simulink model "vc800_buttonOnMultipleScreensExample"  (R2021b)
settings: Solver=FixedStepDiscrete  StartTime=0.0  StopTime=10.0  FixedStep=0.01  RelTol=1e-3  EnableMultiTasking=on
PreLoadFcn:
  | try, model_open; catch, disp('Error occurred while executing model pre-load callback: model_open.m'); disp('Please assure that the MATLAB working directory is set to the model directory before opening.'); end
InitFcn:
  | try, model_open; catch, end
model workspace (MAT data in the model file):
  IOScreen_Label_XCoord = 1
  IOScreen_Row1_YCoord = 1
  IOScreen_Row2_YCoord = 12
  IOScreen_Value_XCoord = 110
  MainScreen_Row1_YCoord = 7
  MainScreen_Row2_YCoord = 23
  MainScreen_Symbols_XCoord = 1
  MainScreen_Units_XCoord = 69
  MainScreen_Value_XCoord = 64
undefined symbols (not defined in the file or in its folder): case, curr_screen, default, DISP, filtering, gesture, hex2dec, Mode, No, raptor_get_buildNum, raptor_get_safe_string, raptor_hwexp, raptor_xcp_function, Screens, VC800, Voltage
libraries: Raptor_display_lib x190, Raptor_lib x97, simulink_extras x11, Raptor_Datalogging_lib x10, simulink x2
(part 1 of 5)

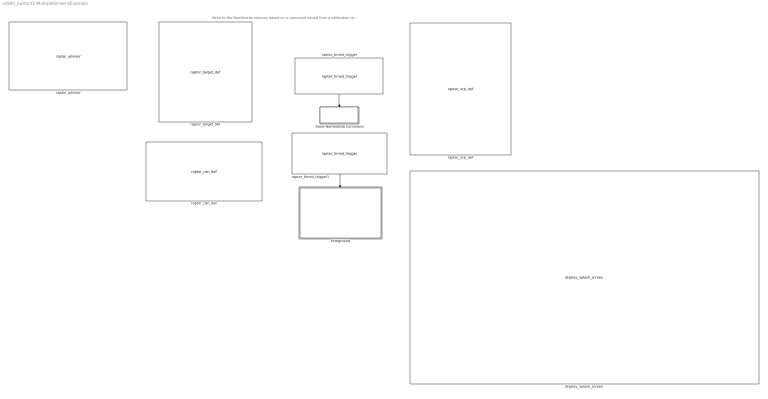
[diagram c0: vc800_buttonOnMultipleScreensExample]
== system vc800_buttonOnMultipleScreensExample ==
  note: Write to the NonVolatile memory based on a command issued from a calibration tool. This display does not have an option for a controlled shutdown but too many writes will burn out the internal NonVolatile memory.
  Foreground : Subsystem
  Store NonVolatile Command : Subsystem  TreatAsAtomicUnit=on
  display_splash_screen : Raptor_display_lib/Screen Functions/display_splash_screen  ImageFile=background_newsplash.bmp
  raptor_advisor : Raptor_lib/Configuration/raptor_advisor  pop_setEnable=Enable All  ckb_Raptor=on  ckb_AppMonitor=on  tbl_AppMonitor={ 'on', 'App Monitor'; 'on', 'App Monitor Measurement'; 'on', 'App Monitor Stop'; 'on', 'Reboot'; 'on', 'Task Monitor'; 'on', 'Task Monitor Measurement' }  ckb_CAN=on  tbl_CAN="{ 'on', 'CAN Baud Rate'; 'on', 'CAN Bus Off Recovery'; 'on', 'CAN Definition'; 'on', 'CAN Hardware Mailbox Config'; 'on', 'CAN Mailbox Properties'; 'on', 'CAN Partial Networking'; 'on', 'CAN Queue Info'; 'on', 'CAN Rx Message'; 'on', 'CAN Rx Raw'; 'on', 'CAN State'; 'on', 'CAN Trigger'; 'on', 'CAN Tx Message'; 'on', 'CAN Tx Raw'; 'on', 'CAN/FD Definition'; 'on', 'CAN/FD Rx Message'; 'on', 'CAN/FD 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"  ckb_Checksum=on  tbl_Checksum={ 'on', 'Calculate Checksum'; 'on', 'Read Checksum' }  ckb_Config=on  tbl_Config={ 'on', 'Configuration Read'; 'on', 'System Variable Access Level'; 'on', 'ECU Definition'; 'on', 'Set Target Address'; 'on', 'XCP Custom Security Seed/Key'; 'on', 'XCP Custom Security Trigger'; 'on', 'XCP Protocol Definition'; 'on', 'XCP Query'; 'on', 'XCP Set Address' }  ckb_DataStore=on  tbl_DataStore={ 'on', 'Adjustment'; 'on', 'Data Store'; 'on', 'Data Read'; 'on', 'Data Write'; 'on', 'Load NonVolatile Defaults'; 'on', 'Fixed NV Manager'; 'on', 'Measurement'; 'on', 'Memory Read'; 'on', 'NonVolatile Settings'; 'on', 'Override'; 'on', 'Fixed NonVolatile Status'; 'on', 'NonVolatile Status'; 'on', 'Store NonVolatile' }  ckb_Engine=on  tbl_Engine={ 'on', 'Angle Time'; 'on', 'CamShaft Sensor Info'; 'on', 'Encoder Def'; 'on', 'Injector Output'; 'on', 'Knock Results'; 'on', 'Knock Input'; 'on', 'Spark Output'; 'on', 'Wideband O2 Input' }  ckb_Ethernet=on  tbl_Ethernet="{ 'on', 'Ethernet Adapter Get MAC Address'; 'on', 'Ethernet Definition'; 'on', 'Ethernet Interface Definition'; 'on', 'Ethernet Interface Get VLAN'; 'on', 'Ethernet Interface Set VLAN'; 'on', 'Ethernet Socket - TCP Server'; 'on', 'Ethernet Socket - UDP Server'; 'on', 'Ethernet Socket State'; 'on', 'Ethernet TCP Accept'; 'on', 'Ethernet TCP Close'; 'on', 'Ethernet TCP Connect'; 'on', 'Ethernet TCP 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"  ckb_OBD_Faults=on  tbl_OBD_Faults={ 'on', 'OBD Counter'; 'on', 'Increment OBD Counter'; 'on', 'Read OBD Counter'; 'on', 'Reset OBD Counter'; 'on', 'Drive Cycle Complete'; 'on', 'OBD Ratio'; 'on', 'Increment OBD Ratio'; 'on', 'Read OBD Ratio'; 'on', 'Reset OBD Ratio' }  ckb_Faults=on  tbl_Faults={ 'on', 'Fault Action'; 'on', 'Fault Action Iterator'; 'on', 'Fault Action Read'; 'on', 'Clear Fault'; 'on', 'Fault Data'; 'on', 'Fault Data Read'; 'on', 'Fault Data Write'; 'on', 'Fault'; 'on', 'Fault Handle'; 'on', 'Fault Iterator'; 'on', 'Fault Manager'; 'on', 'Fault Measurement'; 'on', 'Null Fault'; 'on', 'Fault Config'; 'on', 'Fault Reference'; 'on', 'Set Fault State'; 'on', 'Fault State Iter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  ckb_IO=on  tbl_IO={ 'on', 'Analog Input'; 'on', 'Analog Input Reference'; 'on', 'Analog Output'; 'on', 'Device Diagnostics'; 'on', 'Digital Input'; 'on', 'Digital Output'; 'on', 'Frequency Input'; 'on', 'H-Bridge Output'; 'on', 'IMU Calibrate'; 'on', 'IMU Reset'; 'on', 'IMU Status'; 'on', 'Inertial Measurement'; 'on', 'Input Capture Defn'; 'on', 'Input Capture Get'; 'on', 'Input Capture Trigger'; 'on', 'Input Statu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  ckb_LIN=on  tbl_LIN={ 'on', 'LIN Master Definition'; 'on', 'LIN Get Schedule'; 'on', 'LIN Rx Message'; 'on', 'LIN Set Schedule'; 'on', 'LIN Slave Definition'; 'on', 'LIN State'; 'on', 'LIN Trigger'; 'on', 'LIN Tx Message' }  ckb_SENT=on  tbl_SENT={ 'on', 'SENT Definition'; 'on', 'SENT Receive State' }  ckb_Serial=on  tbl_Serial={ 'on', 'Serial Definition'; 'on', 'Serial Rx'; 'on', 'Serial Trigger'; 'on', 'Serial Tx' }  ckb_Strings=on  tbl_Strings={ 'on', 'String'; 'on', 'Arr 2 Str'; 'on', 'String Length'; 'on', 'Printf'; 'on', 'String Reference'; 'on', 'scanf'; 'on', 'Str 2 Arr' }  ckb_Tables=on  tbl_Tables={ 'on', 'Table Adapt'; 'on', 'Axis'; 'on', 'Axis Reference'; 'on', 'Table Interpolate 1D'; 'on', 'Table Interpolate 1D Reference'; 'on', 'Table Interpolate 2D'; 'on', 'Table Interpolate 2D Reference' }  ckb_Time=on  tbl_Time={ 'on', 'Datetime Conversion In'; 'on', 'Datetime Conversion Out'; 'on', 'Real Time Clock Read'; 'on', 'Real Time Clock Set' }  ckb_Triggers=on  tbl_Triggers={ 'on', 'App Trigger'; 'on', 'dT'; 'on', 'Distributed Action Defn'; 'on', 'Distributed Action Execute'; 'on', 'Distributed Action Trigger'; 'on', 'Shutdown'; 'on', 'Sleep'; 'on', 'Startup'; 'on', 'Time'; 'on', 'Timed Trigger'; 'on', 'Timed Trigger Config'; 'on', 'Define Trigger'; 'on', 'Trigger Execute'; 'on', 'Output Trigger Reference'; 'on', 'Trigger Select' }  ckb_DataLog=on  tbl_DataLog={ 'on', 'Data Log Erase'; 'on', 'Data Log Read'; 'on', 'Data Log Write'; 'on', 'File Close'; 'on', 'File EOF'; 'on', 'File Exists'; 'on', 'File Get Free Space'; 'on', 'File Open'; 'on', 'File Position'; 'on', 'File Read'; 'on', 'File Remove'; 'on', 'File Rename'; 'on', 'File Seek'; 'on', 'File Size'; 'on', 'File Sync'; 'on', 'USB Eject'; 'on', 'USB Status'; 'on', 'File Write' }  ckb_Display=on  ckb_Drawing=on  tbl_Drawing={ 'on', 'Clear Rect'; 'on', 'Clear Screen'; 'on', 'Draw Arc'; 'on', 'Draw Button'; 'on', 'Draw Circle'; 'on', 'Draw Image'; 'on', 'Draw Line'; 'on', 'Draw Polygon'; 'on', 'Draw Rectangle'; 'on', 'Draw Text'; 'on', 'Element'; 'on', 'Fill Circle'; 'on', 'Fill Ellipse'; 'on', 'Fill Polygon'; 'on', 'Fill Rect'; 'on', 'Image Ref' }  ckb_Menu=on  tbl_Menu={ 'on', 'Menu Screen Definition'; 'on', 'Menu Sel Item'; 'on', 'Menu Text'; 'on', 'Menu Title' }  ckb_Prefab=on  tbl_Prefab={ 'on', 'Gauge: Create'; 'on', 'Gauge: Update' }  ckb_ScreenFuncs=on  tbl_ScreenFuncs={ 'on', 'Hide Buttonbar'; 'on', 'Button Bar Properties'; 'on', 'Setup Button'; 'on', 'Goto Screen'; 'on', 'Recalibrate Screen'; 'on', 'Screen Definition'; 'on', 'Screen Reference'; 'on', 'Screen Select'; 'on', 'Splash Screen' }  ckb_Touchscreen=on  tbl_Touchscreen={ 'on', 'Button Status'; 'on', 'Display Touchscreen'; 'on', 'Button Def'; 'on', 'Hot Area Actions'; 'on', 'Update Swipe Action' }  ckb_Modbus=on  tbl_Modbus={ 'on', 'Modbus Master'; 'on', 'Modbus Slave'; 'on', 'Modbus Slave Error'; 'on', 'Modbus Slave Response' }  ckb_Routing=on  tbl_Routing={ 'on', 'J1939 Message Router'; 'on', 'Message Hardware Filter'; 'on', 'Message Network'; 'on', 'Message Router' }  ckb_Safe=on  tbl_Safe={ 'on', 'Raptor Stack Check' }  ckb_J1939=on  ckb_DMA=on  tbl_DMA={ 'on', 'DM14/15/16 Definition: DM14 Rx'; 'on', 'DM14/15/16 Definition: DM15 Rx'; 'on', 'DM14/15/16 Definition: DM15 Tx'; 'on', 'DM14/15/16 Definition: DMA Manager'; 'on', 'DMA Address Space Definition'; 'on', 'DMA Address Space Return'; 'on', 'DMA Address Space Trigger'; 'on', 'DMA Key'; 'on', 'DMA Key Trigger' }  ckb_DM_Msgs=on  tbl_DM_Msgs={ 'on', 'DM4 Transmit'; 'on', 'DM5 Transmit'; 'on', 'DM8 Transmit'; 'on', 'DM19 Transmit'; 'on', 'DM20 Transmit'; 'on', 'DM21 Transmit'; 'on', 'DM22 Rx Trigger'; 'on', 'DM24 Transmit'; 'on', 'DM25 Transmit'; 'on', 'DM26 Transmit'; 'on', 'DM29 Transmit'; 'on', 'DM30 Transmit'; 'on', 'DM33 Transmit'; 'on', 'DM34 Transmit'; 'on', 'DTC Transmit' }  ckb_EFF=on  tbl_EFF={ 'on', 'Clear Expanded FF'; 'on', 'Write Expanded FF'; 'on', 'Expanded FF Status' }  ckb_PGN_Tx=on  tbl_PGN_Tx={ 'on', 'CBI Transmit'; 'on', 'CI Transmit'; 'on', 'EC1 Transmit'; 'on', 'ECUID Transmit'; 'on', 'GTFI Transmit'; 'on', 'LTFI Transmit'; 'on', 'RC Transmit'; 'on', 'SOFT Transmit'; 'on', 'TTI2 Transmit'; 'on', 'VI Transmit' }  ckb_SPN=on  tbl_SPN={ 'on', 'SPN Read'; 'on', 'SPN Write' }  ckb_J1939_TP=on  tbl_J1939_TP={ 'on', 'J1939 DTC Rx Handler'; 'on', 'Source Addr'; 'on', 'PGN Enable'; 'on', 'PGN Request Slot'; 'on', 'PGN Enable'; 'on', 'PGN Trigger'; 'on', 'Tx ACK/NACK'; 'on', 'J1939 Protocol'; 'on', 'J1939 Transport Protocol Receive'; 'on', 'PGN Rx Trigger' }  ckb_UDS=on  ckb_ISO14229=on  tbl_ISO14229={ 'on', 'ISO14229 Custom Service 0x31'; 'on', 'ISO14229 Service 0x10 - Session Control'; 'on', 'ISO14229 Service 0x11 - ECU Reset'; 'on', 'ISO14229 Service 0x14 - Clear Diagnostic Information'; 'on', 'ISO14229 Service 0x19 - Read DTC Information'; 'on', 'ISO14229 Service 0x19 - Extended Data Definition'; 'on', 'ISO14229 Service 0x19 - Snapshot Record Definition'; 'on', 'ISO14229 Service 0x19 - Sna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  ckb_ISO15031=on  tbl_ISO15031={ 'on', 'ISO15031 Custom Service'; 'on', 'ISO15031 Service 0x01'; 'on', 'ISO15031 Service 0x03 - Emission-related diagnostic trouble codes'; 'on', 'ISO15031 Service 0x04 - Clear Diagnostic Information'; 'on', 'ISO15031 Service 0x07 - Emission-related pending diagnostic trouble codes'; 'on', 'ISO15031 Service 0x09 - Calibration Identification'; 'on', 'ISO15031 Service 0x09 - Calibration Verificatio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  ckb_ISO15765=on  tbl_ISO15765={ 'on', 'ISO15765 Protocol Receive Queue Info'; 'on', 'ISO15765 Protocol Transmit Queue Info'; 'on', 'ISO15765 Protocol Transmit Raw' }  ckb_UDS_Basics=on  tbl_UDS_Basics={ 'on', 'UDS Client Functional Address Request'; 'on', 'UDS Protocol Client Request Raw'; 'on', 'UDS Protocol Receive Raw'; 'on', 'UDS Server Service Process Raw'; 'on', 'UDS Protocol Transmit Raw' }  ckb_UDS_Other=on  tbl_UDS_Other={ 'on', 'UDS Protocol'; 'on', 'UDS Set Buffer Storage' }
  raptor_can_def : Raptor_lib/CAN/raptor_can_def  canBus='CAN1'  resourceValues=CAN1|(None)  resource=CAN1  baudRateValues=125k|250k|500k|1000k  baudRate=250k  enable_baud_rate_config=0  sim_func_name='ConfigureCANBaudRate'  createButton=[]  txQueueSize=16  rxQueueSize=16  useCustomBR=0  customBR='CustomBaudRate'  updateButton=[]
  raptor_target_def : Raptor_lib/Configuration/raptor_target_def  targetValues=DISP-VC128-1901|DISP-VC320L-1402|DISP-VC320-1204|DISP-VC800-1402|DISP-VC500-1904|DISP-VC700-2003|DISP-VC300R-2004|GCM-5634M-070-1559|GCM-5634M-070-1562|ECM-1793-196-1503|GCM-1793-196-1503|GCM-5605B-048-1906|GCM-5605B-048-2104|RCM-5743R-080-2005|RCM-5743R-080-2106|RCM-5743R-080-2203|RCM-5743R-080-2304|UAS-5743R-047-2102|UAS-5743R-047-2107|EOL-58NN-176-2204|RCM-58NN-112-2103|RCM-58NN-112-2202|RCM-58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  target=DISP-VC800-1402  simpack=0  simulator=1  heap=2*1024  stack=2*1024  fgndStack=2*1024  bgndStack=2*1024  idleStack=1024  intStack=1536  sdStack=1024  appStack=1024  ecuaddr=253  uds_server_addr_ext=0  uds_server_addr=hex2dec('600')  uds_client_addr=hex2dec('650')  callocValues=Constant (FLASH)|NonVolatile (EEPROM)  calloc=NonVolatile (EEPROM)  compilerValues=Device:arm-2014.05_1.0.0 Simulator:None (disabled)|Device:arm-2014.05_1.0.0 Simulator:Visual Studio Community 2017  compiler=Device:arm-2014.05_1.0.0 Simulator:Visual Studio Community 2017  setFileName=1  exeName=[raptor_get_safe_string(bdroot) '_']  addBuildNum=1  minVerChars=3  extraOutput=0  buildLocationValues=Raptor Default|Model Directory|User Defined  buildLocation=Raptor Default  exeLocation=''  exeFileButton=0  a2lLocation=''  a2lFileButton=0  rpgLocation=''  rpgFileButton=0
  raptor_timed_trigger : Raptor_lib/Triggers/raptor_timed_trigger  triggerValues=Foreground|Foregroundx2|Foregroundx5|Foregroundx10|Foregroundx50|Background|Backgroundx2|Backgroundx5|Backgroundx10|Backgroundx20|Second|Minute  trigger=Background  inherited=0  alwaysEnabled=1  triggerPriority=0  triggerName=BGND_kLoVr
  raptor_timed_trigger1 : Raptor_lib/Triggers/raptor_timed_trigger  triggerValues=Foreground|Foregroundx5|Foregroundx10|Foregroundx50|Second|Minute  trigger=Foreground  inherited=0  alwaysEnabled=1  triggerPriority=0  triggerName=7Je7r
  raptor_xcp_def : Raptor_lib/Configuration/raptor_xcp_def  XCPname='XCP1'  canBus='CAN1'  bcID=hex2dec('100')  bcID_TypeValues=Standard|Extended  bcID_Type=Standard  rxID=hex2dec('200')  rxID_TypeValues=Standard|Extended  rxID_Type=Standard  txID=hex2dec('300')  txID_TypeValues=Standard|Extended  txID_Type=Standard  daqRates=[10 100]  numODTs=20  genCANAPE=0  genVISION=0  securityValues=Standard|None|Custom User Defined|MH_SB_4  security=Standard  dllName=raptor_XCPSecurity.dll  accessValues=4|3|2|1  access=1  bcStorageValues=[]  bcStorage=Calibration  txStorageValues=[]  txStorage=Calibration  rxStorageValues=[]  rxStorage=Calibration
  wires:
  raptor_timed_trigger1/1 -> Foreground/Trigger
  raptor_timed_trigger/1 -> Store NonVolatile Command/Trigger

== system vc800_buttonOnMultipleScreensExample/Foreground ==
  Trigger : TriggerPort  TriggerType=function-call  VariantControl=Variant  PortDimensions=1
  Display : Subsystem
  Plant : Subsystem
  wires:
  Display/1(Actuators) -> Plant/1(Actuators)
  Plant/1(Sensors) -> Display/1(Sensors)

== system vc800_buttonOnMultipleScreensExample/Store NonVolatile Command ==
  note: Setting the StoreNonvolatileCommand value to to 1 in the calibration tool will cause this subsystem to execute, calling the 'Store Nonvolatile' function. The StoreNonvolatileCommand value will be set to 0 inside the subsytem so that the Store event happens once.
  function : TriggerPort  TriggerType=function-call  VariantControl=Variant
  Store NV : Subsystem  TreatAsAtomicUnit=on
  raptor_data_def : Raptor_lib/Data Storage/raptor_data_def  dataName='StoreNonVolatileCommand'  initValue=false  dataType=boolean  storage=Volatile (RAM)  calVisible=on  calType=Adjustment  calDispType=Enumeration  calEnum={'Not Writing', 'Start Write'}  calGain=1.0  calOffset=0  calMin=-inf  calMax=inf  calFormat='-1'  calUnit=''  calHelp=''  calAccess=1  calFunction=raptor_xcp_function(gcb)  calDispHeaders=off  calColHeaders={'Col1' 'Col2' 'Col3'}  calRowHeaders={'Row1' 'Row2' 'Row3'}
  raptor_data_read : Raptor_lib/Data Storage/raptor_data_read  dataName='StoreNonVolatileCommand'  dataShape=Scalar  idxSource=Input  idxRow=1  idxCol=1
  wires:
  raptor_data_read/1 -> Store NV/Enable

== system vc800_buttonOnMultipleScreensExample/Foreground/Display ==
  Sensors : Inport
  Data Logging : Subsystem
  Screens : Subsystem
  Unit Delay : UnitDelay  SampleTime=-1  HasFrameUpgradeWarning=on
  Actuators : Outport  VectorParamsAs1DForOutWhenUnconnected=off
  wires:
  Sensors/1 -> Data Logging/2(In Bus Element8), Screens/1(Sensors)
  Screens/1(ActuatorCommands) -> Actuators/1
  Screens/2(Out Bus Element) -> Data Logging/1(In Bus Element4)
  Data Logging/1(Out Bus Element) -> Unit Delay/1
  Unit Delay/1 -> Screens/2(DataLogState)

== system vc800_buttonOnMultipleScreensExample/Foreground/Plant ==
  Actuators : Inport
  Inputs : Subsystem
  Outputs : Subsystem
  Sensors : Outport  VectorParamsAs1DForOutWhenUnconnected=off
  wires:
  Actuators/1 -> Outputs/1(In Bus Element)
  Inputs/1(Out Bus Element2) -> Sensors/1

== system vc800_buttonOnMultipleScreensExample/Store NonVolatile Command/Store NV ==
  Enable : EnablePort
  Constant : Constant  Value=false
  Function-Call Generator : simulink/Ports & Subsystems/Function-Call Generator  sample_time=-1  numberOfIterations=1  DisallowWideOutput=off
  raptor_data_write : Raptor_lib/Data Storage/raptor_data_write  dataName='StoreNonVolatileCommand'  dataShape=Scalar  idxSource=Input Port  idxRow=1  idxCol=1
  raptor_store_nv : Raptor_lib/Data Storage/raptor_store_nv  null=0
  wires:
  Function-Call Generator/1 -> raptor_store_nv/Trigger
  Constant/1 -> raptor_data_write/1

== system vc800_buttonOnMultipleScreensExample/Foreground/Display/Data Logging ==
  In Bus Element4 : Inport
  In Bus Element{,1..3,5..8} (8 alike) : Inport  Port=2
  Bus Creator : BusCreator  Inputs=4
  Logical Operator : Logic  AllPortsSameDT=off  OutDataTypeStr=boolean
  Write to Log : Subsystem
  raptor_data_read1 : Raptor_lib/Data Storage/raptor_data_read  dataName='LogCounter'  dataShape=Scalar  idxSource=Input  idxRow=1  idxCol=1
  raptor_measurement : Raptor_lib/Data Storage/raptor_measurement  paramName='USBInserted'  nameSource=Parameter  calDispType=Number  calEnum={'False', 'True'}  calGain=1.0  calOffset=0.0  calMax=inf  calMin=-inf  calFormat='-1'  calUnit=''  calHelp=''  calAccess=1  calFunction=raptor_xcp_function(gcb)  calVisible=on
  raptor_measurement1 : Raptor_lib/Data Storage/raptor_measurement  paramName='EjectReady'  nameSource=Parameter  calDispType=Number  calEnum={'False', 'True'}  calGain=1.0  calOffset=0.0  calMax=inf  calMin=-inf  calFormat='-1'  calUnit=''  calHelp=''  calAccess=1  calFunction=raptor_xcp_function(gcb)  calVisible=on
  raptor_measurement3 : Raptor_lib/Data Storage/raptor_measurement  paramName='LoggingReady'  nameSource=Parameter  calDispType=Number  calEnum={'False', 'True'}  calGain=1.0  calOffset=0.0  calMax=inf  calMin=-inf  calFormat='-1'  calUnit=''  calHelp=''  calAccess=1  calFunction=raptor_xcp_function(gcb)  calVisible=on
  Out Bus Element{,1..4} (5 alike) : Outport  VectorParamsAs1DForOutWhenUnconnected=off
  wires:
  In Bus Element/1 -> raptor_measurement/1, Out Bus Element4/1  "USBInserted"
  Bus Creator/1 -> Write to Log/1(data)
  In Bus Element1/1 -> raptor_measurement1/1, Out Bus Element3/1
  In Bus Element2/1 -> Write to Log/2(drive)
  In Bus Element3/1 -> raptor_measurement3/1, Out Bus Element/1, Logical Operator/1
  Logical Operator/1 -> Out Bus Element1/1, Write to Log/Enable  "LoggingActive"
  raptor_data_read1/1 -> Out Bus Element2/1
  In Bus Element4/1 -> Logical Operator/2
  In Bus Element5/1 -> Bus Creator/1
  In Bus Element6/1 -> Bus Creator/2
  In Bus Element7/1 -> Bus Creator/3
  In Bus Element8/1 -> Bus Creator/4

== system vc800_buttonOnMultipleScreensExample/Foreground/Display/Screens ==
  note: The button also needs Draw Button blocks placed in the Update Screen functions for all screens it should appear on.
  note: This triggered subsystem defines what the button does.
  note: This button is defined once.
  Sensors : Inport
  DataLogState : Inport  Port=2
  AboutScreen_Create : Subsystem  TreatAsAtomicUnit=on
  AboutScreen_Update : Subsystem  TreatAsAtomicUnit=on
  Bus Creator : BusCreator  Inputs=2
  DataLogScreen_Create : Subsystem  TreatAsAtomicUnit=on
  DataLogScreen_CurrentScreen : Subsystem  TreatAsAtomicUnit=on
  DataLogScreen_Update : Subsystem  TreatAsAtomicUnit=on
  Display Button Status : Raptor_display_lib/Touchscreen/Display Button Status  ButtonName='GoToAbout'
  Go_To_About_Screen : Subsystem
  InputScreen_Create : Subsystem  TreatAsAtomicUnit=on
  InputScreen_Update : Subsystem  TreatAsAtomicUnit=on
  MainScreen_Create : Subsystem  TreatAsAtomicUnit=on
  MainScreen_Update : Subsystem  TreatAsAtomicUnit=on
  Navigation : Subsystem
  OutputScreen_Create : Subsystem  TreatAsAtomicUnit=on
  OutputScreen_Update : Subsystem  TreatAsAtomicUnit=on
  Terminator{,1..6,19} (8 alike) : Terminator
  display_button_def : Raptor_display_lib/Touchscreen/display_button_def  ButtonName='GoToAbout'  ImageFile='blank.png'  PressedImageFile='blank_s.png'  font=Arial  fontFile=''  TextLine1='About'  HeightLine1=12  TextLine2='Screen'  HeightLine2=12  TextUnderButton=''  HeightUnderButton=12  buttonMargin=0  underMargin=0  buttonVAlign=Center  underVAlign=Center  buttonHAlign=Center  underHAlign=Center  underSide=Bottom  col='0000'  pressedCol='07E0'  underCol='0000'  pressedUnderCol='07E0'
  display_screen_definition : Raptor_display_lib/Screen Functions/display_screen_definition  ScreenName='MainScreen'  selectAtInit=true  useSimFuncs=off  useInitFunc=on  init_func_name=''  useCreateFunc=on  bgnd_func_name=''  useUpdateFunc=on  fgnd_func_name=''
  display_screen_definition1 : Raptor_display_lib/Screen Functions/display_screen_definition  ScreenName='InputScreen'  selectAtInit=false  useSimFuncs=off  useInitFunc=on  init_func_name=''  useCreateFunc=on  bgnd_func_name=''  useUpdateFunc=on  fgnd_func_name=''
  display_screen_definition2 : Raptor_display_lib/Screen Functions/display_screen_definition  ScreenName='AboutScreen'  selectAtInit=false  useSimFuncs=off  useInitFunc=on  init_func_name=''  useCreateFunc=on  bgnd_func_name=''  useUpdateFunc=on  fgnd_func_name=''
  display_screen_definition3 : Raptor_display_lib/Screen Functions/display_screen_definition  ScreenName='DataLogScreen'  selectAtInit=false  useSimFuncs=off  useInitFunc=on  init_func_name=''  useCreateFunc=on  bgnd_func_name=''  useUpdateFunc=on  fgnd_func_name=''
  display_screen_definition4 : Raptor_display_lib/Screen Functions/display_screen_definition  ScreenName='OutputScreen'  selectAtInit=false  useSimFuncs=off  useInitFunc=on  init_func_name=''  useCreateFunc=on  bgnd_func_name=''  useUpdateFunc=on  fgnd_func_name=''
  ActuatorCommands : Outport  VectorParamsAs1DForOutWhenUnconnected=off
  Out Bus Element : Outport  Port=2  VectorParamsAs1DForOutWhenUnconnected=off
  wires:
  display_screen_definition/1 -> Terminator2/1
  display_screen_definition/2 -> MainScreen_Create/Trigger
  display_screen_definition/3 -> MainScreen_Update/Trigger
  display_screen_definition/4 -> Terminator/1
  OutputScreen_Update/1(Actuators) -> Bus Creator/2
  Bus Creator/1 -> ActuatorCommands/1
  display_screen_definition2/1 -> Terminator1/1
  display_screen_definition2/3 -> AboutScreen_Update/Trigger
  display_screen_definition2/2 -> AboutScreen_Create/Trigger
  display_screen_definition2/4 -> Terminator5/1
  display_screen_definition3/4 -> DataLogScreen_CurrentScreen/Enable
  display_screen_definition3/2 -> DataLogScreen_Create/Trigger
  display_screen_definition3/3 -> DataLogScreen_Update/Trigger
  display_screen_definition3/1 -> Terminator3/1
  DataLogScreen_Update/1(Commands) -> Out Bus Element/1
  DataLogState/1 -> DataLogScreen_Update/2(DataLogState)
  Sensors/1 -> InputScreen_Update/1(Sensors), DataLogScreen_Update/1(Sensors), Bus Creator/1, MainScreen_Update/1(In Bus Element)
  display_screen_definition4/2 -> OutputScreen_Create/Trigger
  display_screen_definition4/3 -> OutputScreen_Update/Trigger
  display_screen_definition1/2 -> InputScreen_Create/Trigger
  display_screen_definition1/1 -> Terminator19/1
  display_screen_definition4/4 -> Terminator6/1
  display_screen_definition1/3 -> InputScreen_Update/Trigger
  display_screen_definition1/4 -> Terminator4/1
  Display Button Status/1 -> Go_To_About_Screen/Trigger

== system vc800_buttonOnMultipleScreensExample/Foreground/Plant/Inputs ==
  Inputs : Subsystem
  J1939 Rx : Subsystem
  USB : Subsystem
  Out Bus Element{1..27} (27 alike) : Outport  VectorParamsAs1DForOutWhenUnconnected=off
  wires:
  J1939 Rx/1(Engine RPM) -> Out Bus Element2/1
  J1939 Rx/2(Engine RPM Valid) -> Out Bus Element3/1
  J1939 Rx/3(Illumination) -> Out Bus Element4/1
  J1939 Rx/4(Illumination1) -> Out Bus Element5/1
  USB/1(USBInserted) -> Out Bus Element1/1
  USB/2(USBEjectReady) -> Out Bus Element6/1
  USB/3(USBPath) -> Out Bus Element7/1
  USB/4(USBReadyToLog) -> Out Bus Element8/1
  USB/5(USBFreeSpace) -> Out Bus Element9/1
  Inputs/18(Input18) -> Out Bus Element27/1
  Inputs/2(Input2) -> Out Bus Element11/1
  Inputs/13(Input13) -> Out Bus Element22/1
  Inputs/14(Input14) -> Out Bus Element23/1
  Inputs/12(Input12) -> Out Bus Element21/1
  Inputs/11(Input11) -> Out Bus Element20/1
  Inputs/4(Input4) -> Out Bus Element13/1
  Inputs/1(Input1) -> Out Bus Element10/1
  Inputs/5(Input5) -> Out Bus Element14/1
  Inputs/9(Input9) -> Out Bus Element18/1
  Inputs/8(Input8) -> Out Bus Element17/1
  Inputs/16(Input16) -> Out Bus Element25/1
  Inputs/17(Input17) -> Out Bus Element26/1
  Inputs/6(Input6) -> Out Bus Element15/1
  Inputs/7(Input7) -> Out Bus Element16/1
  Inputs/3(Input3) -> Out Bus Element12/1
  Inputs/15(Input15) -> Out Bus Element24/1
  Inputs/10(Input10) -> Out Bus Element19/1

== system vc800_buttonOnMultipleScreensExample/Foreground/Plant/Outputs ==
  In Bus Element{,2..11} (11 alike) : Inport
  Constant : Constant  OutDataTypeStr=uint32
  Data Type Conversion : DataTypeConversion  OutDataTypeStr=uint16
  Gain : Gain  Gain=100  OutDataTypeStr=single  RndMeth=Simplest  SaturateOnIntegerOverflow=on
  Outputs : Subsystem
  raptor_digital_out6 : Raptor_lib/Input & Output/raptor_digital_out  resourceValues=OUTPUT1|BUZZER_MUTE|BUZZER|(None)  resource=BUZZER_MUTE  driverTypeValues=Internal  driverType=Internal
  raptor_digital_out7 : Raptor_lib/Input & Output/raptor_digital_out  resourceValues=OUTPUT1|BUZZER_MUTE|BUZZER|(None)  resource=BUZZER  driverTypeValues=Internal  driverType=Internal
  raptor_pwm_out : Raptor_lib/Input & Output/raptor_pwm_out  showEnable=0  resourceValues=OUTPUT1|LED1|LED2|LED3|LED4|LCD_BACKLIGHT|KEYPAD_BACKLIGHT|(None)  resource=LCD_BACKLIGHT  driverTypeValues=LED  driverType=LED
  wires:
  In Bus Element/1 -> Gain/1
  Gain/1 -> Data Type Conversion/1
  Data Type Conversion/1 -> raptor_pwm_out/1
  Constant/1 -> raptor_pwm_out/2
  In Bus Element2/1 -> raptor_digital_out7/1
  In Bus Element3/1 -> raptor_digital_out6/1
  In Bus Element8/1 -> Outputs/5(Output5)
  In Bus Element4/1 -> Outputs/1(Output1)
  In Bus Element11/1 -> Outputs/8(Output8)
  In Bus Element6/1 -> Outputs/3(Output3)
  In Bus Element7/1 -> Outputs/4(Output4)
  In Bus Element9/1 -> Outputs/6(Output6)
  In Bus Element10/1 -> Outputs/7(Output7)
  In Bus Element5/1 -> Outputs/2(Output2)

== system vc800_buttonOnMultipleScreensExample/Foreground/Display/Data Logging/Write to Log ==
  data : Inport
  drive : Inport  Port=2
  Enable : EnablePort
  Create New File : Subsystem  TreatAsAtomicUnit=on
  File Write Action : Subsystem
  If : If  IfExpression=u1
  Merge : Merge
  Merge1 : Merge
  Open Existing File : Subsystem  TreatAsAtomicUnit=on
  raptor_fileIO_exists1 : Raptor_Datalogging_lib/raptor_fileIO_exists  resourceValues=Data|USB|(None)  resource=USB
  raptor_measurement1 : Raptor_lib/Data Storage/raptor_measurement  paramName='FileOpen_Success'  nameSource=Parameter  calDispType=Number  calEnum={'False', 'True'}  calGain=1.0  calOffset=0.0  calMax=inf  calMin=-inf  calFormat='4.2'  calUnit=''  calHelp=''  calAccess=4  calFunction=raptor_xcp_function(gcb)  calVisible=on
  raptor_string1 : Raptor_lib/Strings/raptor_string  stringName='LogFileName'  string=''  dynamicSize=Fixed Size  strSize=125  storage=Volatile (RAM)  calVisible=on  calAccess=4  strFunction=raptor_xcp_function(gcb)
  raptor_string_printf : Raptor_lib/Strings/raptor_string_printf  formatString='%s/log.txt'
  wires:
  drive/1 -> raptor_string_printf/2
  Merge1/1 -> raptor_measurement1/1, File Write Action/Enable
  raptor_string1/1 -> raptor_string_printf/1
  raptor_string_printf/1 -> raptor_fileIO_exists1/1, Create New File/1(Path), Open Existing File/1(Path)
  raptor_fileIO_exists1/1 -> If/1
  If/1 -> Open Existing File/Action
  If/2 -> Create New File/Action
  Open Existing File/1(Handle) -> Merge/1
  Create New File/1(Handle) -> Merge/2
  Open Existing File/2(Sucess) -> Merge1/1
  Create New File/2(Success) -> Merge1/2
  data/1 -> File Write Action/1(In Bus Element2)
  Merge/1 -> File Write Action/2(In2)

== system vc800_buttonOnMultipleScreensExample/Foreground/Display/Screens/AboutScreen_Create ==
  function : TriggerPort  TriggerType=function-call  VariantControl=Variant
  AboutScreenSwipe : Subsystem
  Constant16 : Constant  Value=400  OutDataTypeStr=int32
  Constant2 : Constant  Value=440  OutDataTypeStr=int32
  Constant3 : Constant  OutDataTypeStr=int32
  Constant4 : Constant  OutDataTypeStr=int32
  Constant5 : Constant  OutDataTypeStr=int32
  Constant6 : Constant  Value=207  OutDataTypeStr=int32
  display_clear_screen : Raptor_display_lib/Drawing Functions/display_clear_screen  Priority=100  colorPort=off  l1Color=0000  l2Color=FFFF  pnPort=off
  display_draw_image : Raptor_display_lib/Drawing Functions/display_draw_image  imagePort=off  imageFile=top corner logo.png  opacityPort=off  opacity=100  drawMode=Draw Entire Image  alpha=Draw as Transparent  layer=Background  drawModeXY=Top Left  pnPort=off
  display_draw_image1 : Raptor_display_lib/Drawing Functions/display_draw_image  imagePort=off  imageFile=swipe_right_left.png  opacityPort=off  opacity=100  drawMode=Draw Entire Image  alpha=Draw as Transparent  layer=Foreground  drawModeXY=Top Left  pnPort=off
  display_draw_text : Raptor_display_lib/Drawing Functions/display_draw_text  textPort=off  textVal='About'  colorPort=off  col=FFFF  opacity=100  font=Future  fontFile=''  heightPort=off  height=40  hAlign=Center  vAlign=Center  spacing=0  layer=Background  pnPort=off
  raptor_display_swipe_action2 : Raptor_display_lib/Touchscreen/raptor_display_swipe_action  gest_callback_sim_func_name='AboutScreenSwipe'
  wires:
  Constant16/1 -> display_draw_text/1
  Constant2/1 -> display_draw_text/2
  Constant4/1 -> display_draw_image/1
  Constant3/1 -> display_draw_image/2
  Constant6/1 -> display_draw_image1/1
  Constant5/1 -> display_draw_image1/2

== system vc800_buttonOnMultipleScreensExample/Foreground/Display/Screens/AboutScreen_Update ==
  function : TriggerPort  TriggerType=function-call  VariantControl=Variant
  AboutElement : Subsystem
  display_element1 : Raptor_display_lib/Drawing Functions/display_element  colorPort=off  col=0000  layer=Background  pnPort=off
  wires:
  display_element1/1 -> AboutElement/Trigger

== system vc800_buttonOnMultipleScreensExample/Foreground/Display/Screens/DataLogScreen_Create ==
  function : TriggerPort  TriggerType=function-call  VariantControl=Variant
  Button : Raptor_display_lib/Prefab/Button  ButtonName='EjectButtonScreen'  ImageFile='eject_button.png'  PressedImageFile='eject_button_pressed.png'  font=Arial  fontFile=''  TextLine1=''  HeightLine1=12  TextLine2=''  HeightLine2=12  TextUnderButton=''  HeightUnderButton=12  buttonMargin=0  underMargin=0  buttonVAlign=Center  underVAlign=Center  buttonHAlign=Center  underHAlign=Center  underSide=Bottom  col='0000'  pressedCol='07E0'  underCol='0000'  pressedUnderCol='07E0'
  Constant1 : Constant  OutDataTypeStr=int32
  Constant16 : Constant  Value=400  OutDataTypeStr=int32
  Constant2 : Constant  Value=440  OutDataTypeStr=int32
  Constant3 : Constant  OutDataTypeStr=int32
  Constant4 : Constant  OutDataTypeStr=int32
  Constant5 : Constant  Value=150  OutDataTypeStr=int32
  Constant6 : Constant  Value=600 - 35  OutDataTypeStr=int32
  Constant7 : Constant  Value=207  OutDataTypeStr=int32
  DataLogScreenSwipe : Subsystem
  display_clear_screen : Raptor_display_lib/Drawing Functions/display_clear_screen  Priority=100  colorPort=off  l1Color=0000  l2Color=FFFF  pnPort=off
  display_draw_image : Raptor_display_lib/Drawing Functions/display_draw_image  imagePort=off  imageFile=top corner logo.png  opacityPort=off  opacity=100  drawMode=Draw Entire Image  alpha=Draw as Transparent  layer=Background  drawModeXY=Top Left  pnPort=off
  display_draw_image1 : Raptor_display_lib/Drawing Functions/display_draw_image  imagePort=off  imageFile=swipe_right_left.png  opacityPort=off  opacity=100  drawMode=Draw Entire Image  alpha=Draw as Transparent  layer=Foreground  drawModeXY=Top Left  pnPort=off
  display_draw_text : Raptor_display_lib/Drawing Functions/display_draw_text  textPort=off  textVal='Data Logging'  colorPort=off  col=FFFF  opacity=100  font=Future  fontFile=''  heightPort=off  height=40  hAlign=Center  vAlign=Center  spacing=0  layer=Background  pnPort=off
  raptor_display_swipe_action1 : Raptor_display_lib/Touchscreen/raptor_display_swipe_action  gest_callback_sim_func_name='DataLogScreenSwipe'
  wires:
  Constant3/1 -> display_draw_image/2
  Constant4/1 -> display_draw_image/1
  Constant2/1 -> display_draw_text/2
  Constant16/1 -> display_draw_text/1
  Constant5/1 -> Button/2
  Constant6/1 -> Button/1
  Constant7/1 -> display_draw_image1/1
  Constant1/1 -> display_draw_image1/2

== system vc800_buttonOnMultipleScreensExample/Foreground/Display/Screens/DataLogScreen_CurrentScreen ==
  Enable : EnablePort
  Display Button Status1 : Raptor_display_lib/Touchscreen/Display Button Status  ButtonName='EjectButtonScreen'
  EjectButtonPressed : Subsystem
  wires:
  Display Button Status1/1 -> EjectButtonPressed/Trigger

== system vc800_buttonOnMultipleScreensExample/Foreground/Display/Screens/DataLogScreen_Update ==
  Sensors : Inport
  DataLogState : Inport  Port=2
  function : TriggerPort  TriggerType=function-call  VariantControl=Variant
  Element : Subsystem
  display_element1 : Raptor_display_lib/Drawing Functions/display_element  colorPort=off  col=0000  layer=Background  pnPort=off
  Commands : Outport  VectorParamsAs1DForOutWhenUnconnected=off
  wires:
  display_element1/1 -> Element/Trigger
  Element/1(LoggingEnabled) -> Commands/1
  DataLogState/1 -> Element/1(In Bus Element2)
  Sensors/1 -> Element/2(In Bus Element7)

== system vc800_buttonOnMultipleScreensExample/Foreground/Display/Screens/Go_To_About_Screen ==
  Trigger : TriggerPort  VariantControl=(inherit)  PortDimensions=1
  display_goto_screen : Raptor_display_lib/Screen Functions/display_goto_screen  screenPort=off  ScreenName='AboutScreen'

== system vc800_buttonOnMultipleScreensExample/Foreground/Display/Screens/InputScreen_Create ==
  function : TriggerPort  TriggerType=function-call  VariantControl=Variant
  Constant16 : Constant  Value=400  OutDataTypeStr=int32
  Constant2 : Constant  Value=440  OutDataTypeStr=int32
  Constant3 : Constant  OutDataTypeStr=int32
  Constant4 : Constant  OutDataTypeStr=int32
  Constant5 : Constant  OutDataTypeStr=int32
  Constant6 : Constant  Value=207  OutDataTypeStr=int32
  InputScreenSwipe : Subsystem
  display_clear_screen : Raptor_display_lib/Drawing Functions/display_clear_screen  Priority=100  colorPort=off  l1Color=0000  l2Color=FFFF  pnPort=off
  display_draw_image : Raptor_display_lib/Drawing Functions/display_draw_image  imagePort=off  imageFile=top corner logo.png  opacityPort=off  opacity=100  drawMode=Draw Entire Image  alpha=Draw as Transparent  layer=Background  drawModeXY=Top Left  pnPort=off
  display_draw_image1 : Raptor_display_lib/Drawing Functions/display_draw_image  imagePort=off  imageFile=swipe_right_left.png  opacityPort=off  opacity=100  drawMode=Draw Entire Image  alpha=Draw as Transparent  layer=Foreground  drawModeXY=Top Left  pnPort=off
  display_draw_text : Raptor_display_lib/Drawing Functions/display_draw_text  textPort=off  textVal='Inputs'  colorPort=off  col=FFFF  opacity=100  font=Future  fontFile=''  heightPort=off  height=40  hAlign=Center  vAlign=Center  spacing=0  layer=Background  pnPort=off
  raptor_display_swipe_action2 : Raptor_display_lib/Touchscreen/raptor_display_swipe_action  gest_callback_sim_func_name='InputScreenSwipe'
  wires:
  Constant2/1 -> display_draw_text/2
  Constant16/1 -> display_draw_text/1
  Constant4/1 -> display_draw_image/1
  Constant3/1 -> display_draw_image/2
  Constant5/1 -> display_draw_image1/2
  Constant6/1 -> display_draw_image1/1

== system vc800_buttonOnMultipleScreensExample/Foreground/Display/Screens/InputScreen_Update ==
  Sensors : Inport
  function : TriggerPort  TriggerType=function-call  VariantControl=Variant
  InputElement : Subsystem
  display_element1 : Raptor_display_lib/Drawing Functions/display_element  colorPort=off  col=0000  layer=Background  pnPort=off
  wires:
  display_element1/1 -> InputElement/Trigger
  Sensors/1 -> InputElement/1(In Bus Element1)

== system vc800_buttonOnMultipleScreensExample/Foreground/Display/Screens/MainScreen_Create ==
  function : TriggerPort  TriggerType=function-call  VariantControl=Variant
  Constant16 : Constant  Value=400  OutDataTypeStr=int32
  Constant2 : Constant  Value=440  OutDataTypeStr=int32
  Constant3 : Constant  OutDataTypeStr=int32
  Constant4 : Constant  OutDataTypeStr=int32
  Constant5 : Constant  OutDataTypeStr=int32
  Constant6 : Constant  Value=207  OutDataTypeStr=int32
  MainScreenSwipe : Subsystem
  display_clear_screen : Raptor_display_lib/Drawing Functions/display_clear_screen  Priority=100  colorPort=off  l1Color=0000  l2Color=FFFF  pnPort=off
  display_draw_image : Raptor_display_lib/Drawing Functions/display_draw_image  imagePort=off  imageFile=top corner logo.png  opacityPort=off  opacity=100  drawMode=Draw Entire Image  alpha=Draw as Transparent  layer=Background  drawModeXY=Top Left  pnPort=off
  display_draw_image1 : Raptor_display_lib/Drawing Functions/display_draw_image  imagePort=off  imageFile=swipe_right_left.png  opacityPort=off  opacity=100  drawMode=Draw Entire Image  alpha=Draw as Transparent  layer=Foreground  drawModeXY=Top Left  pnPort=off
  display_draw_text : Raptor_display_lib/Drawing Functions/display_draw_text  textPort=off  textVal='J1939'  colorPort=off  col=FFFF  opacity=100  font=Future  fontFile=''  heightPort=off  height=40  hAlign=Center  vAlign=Center  spacing=0  layer=Background  pnPort=off
  raptor_display_swipe_action1 : Raptor_display_lib/Touchscreen/raptor_display_swipe_action  gest_callback_sim_func_name='MainScreenSwipe'
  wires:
  Constant2/1 -> display_draw_text/2
  Constant16/1 -> display_draw_text/1
  Constant4/1 -> display_draw_image/1
  Constant3/1 -> display_draw_image/2
  Constant6/1 -> display_draw_image1/1
  Constant5/1 -> display_draw_image1/2

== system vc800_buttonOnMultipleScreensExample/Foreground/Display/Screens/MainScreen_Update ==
  note: This Draw Button block shows the button on the screen. A button can only be drawn once per screen.
  In Bus Element{,1..3} (4 alike) : Inport
  function : TriggerPort  TriggerType=function-call  VariantControl=Variant
  Add : Sum
  Add1 : Sum
  Brightness Gauge : Raptor_display_lib/Prefab/Gauge  Min=0  Max=100  ScaleValue=1  Dir=Clockwise  StartAngle=-135  StopAngle=135  Scale=150  GaugeFontSize=15  LargeMark=5  SmallMark=2  ArcEnable=off  NeedleColor=EF7D  MarkerColor=FFFF  Image=mgaugeBlk.bmp  imageXOffset=0  imageYOffset=0
  Constant : Constant  Value=390  OutDataTypeStr=Inherit: Inherit via back propagation
  Constant1 : Constant  Value=240  OutDataTypeStr=int32
  Constant2 : Constant  Value=600  OutDataTypeStr=int32
  Constant3 : Constant  Value=100  OutDataTypeStr=int32
  Constant4 : Constant  Value=100  OutDataTypeStr=int32
  Constant5 : Constant  Value=720  OutDataTypeStr=Inherit: Inherit via back propagation
  Constant68 : Constant  Value=240  OutDataTypeStr=int32
  Constant74 : Constant  Value=200  OutDataTypeStr=int32
  Data Type Conversion1 : DataTypeConversion
  Data Type Conversion11 : DataTypeConversion
  Data Type Conversion2 : DataTypeConversion
  Gauge : Raptor_display_lib/Prefab/Gauge  Min=0  Max=8000  ScaleValue=1  Dir=Clockwise  StartAngle=-135  StopAngle=135  Scale=150  GaugeFontSize=15  LargeMark=5  SmallMark=2  ArcEnable=off  NeedleColor=EF7D  MarkerColor=FFFF  Image=mgaugeBlk.bmp  imageXOffset=0  imageYOffset=0
  Ground1 : Ground
  Ground4 : Ground
  Illumination Invalid : Subsystem  TreatAsAtomicUnit=on
  Logical Operator : Logic  Operator=NOT  AllPortsSameDT=off  OutDataTypeStr=boolean
  Logical Operator1 : Logic  Operator=NOT  AllPortsSameDT=off  OutDataTypeStr=boolean
  RPM Invalid : Subsystem  TreatAsAtomicUnit=on
  Terminator : Terminator
  Terminator1 : Terminator
  display_draw_button : Raptor_display_lib/Drawing Functions/display_draw_button  ButtonName='GoToAbout'
  display_draw_text1 : Raptor_display_lib/Drawing Functions/display_draw_text  textPort=off  textVal='Brightness'  colorPort=off  col=FFFF  opacity=100  font=Future  fontFile=''  heightPort=off  height=20  hAlign=Center  vAlign=Center  spacing=0  layer=Background  pnPort=on
  display_draw_text8 : Raptor_display_lib/Drawing Functions/display_draw_text  textPort=off  textVal='RPM'  colorPort=off  col=FFFF  opacity=100  font=Future  fontFile=''  heightPort=off  height=20  hAlign=Center  vAlign=Center  spacing=0  layer=Background  pnPort=on
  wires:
  Constant68/1 -> Add/1, RPM Invalid/2(Ybase), Gauge/3
  In Bus Element/1 -> Data Type Conversion11/1
  Data Type Conversion11/1 -> Gauge/4
  Ground4/1 -> Gauge/1
  Gauge/1 -> RPM Invalid/3(Prev), display_draw_text8/1
  Ground1/1 -> Brightness Gauge/1
  Data Type Conversion1/1 -> Brightness Gauge/4
  In Bus Element2/1 -> Data Type Conversion1/1
  In Bus Element1/1 -> Logical Operator/1
  Logical Operator/1 -> RPM Invalid/Enable
  Logical Operator1/1 -> Illumination Invalid/Enable
  In Bus Element3/1 -> Data Type Conversion2/1
  Data Type Conversion2/1 -> Logical Operator1/1
  display_draw_text8/1 -> Terminator/1
  Constant74/1 -> RPM Invalid/1(Xbase), display_draw_text8/2, Gauge/2
  Constant4/1 -> Add/2
  Add/1 -> display_draw_text8/3
  Add1/1 -> display_draw_text1/3
  Constant3/1 -> Add1/2
  Constant2/1 -> Illumination Invalid/1(Xbase), display_draw_text1/2, Brightness Gauge/2
  display_draw_text1/1 -> Terminator1/1
  Brightness Gauge/1 -> display_draw_text1/1, Illumination Invalid/3(Prev)
  Constant1/1 -> Add1/1, Illumination Invalid/2(Ybase), Brightness Gauge/3
  Constant/1 -> display_draw_button/2
  Constant5/1 -> display_draw_button/1

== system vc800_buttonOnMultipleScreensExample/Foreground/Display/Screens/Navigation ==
  Navigation : TriggerPort  TriggerType=function-call  IsSimulinkFunction=on  FunctionName=Navigation  FunctionVisibility=scoped  VariantControl=Variant  PortDimensions=1
  Go Left : Subsystem  TreatAsAtomicUnit=on
  Go Right : Subsystem  TreatAsAtomicUnit=on
  Go Up or Down : Subsystem  TreatAsAtomicUnit=on
  If : If  IfExpression=u1 == 3  ElseIfExpressions=u1 == 2
  gesture : ArgIn  OutDataTypeStr=uint8  ArgumentName=gesture
  curr_screen : ArgIn  Port=2  OutDataTypeStr=uint8  ArgumentName=curr_screen
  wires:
  curr_screen/1 -> Go Right/1(Current Screen), Go Left/1(Current Screen), Go Up or Down/1(Current Screen)
  If/3 -> Go Up or Down/Action
  gesture/1 -> If/1
  If/2 -> Go Left/Action
  If/1 -> Go Right/Action

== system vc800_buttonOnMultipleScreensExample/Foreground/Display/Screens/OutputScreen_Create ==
  function : TriggerPort  TriggerType=function-call  VariantControl=Variant
  Constant16 : Constant  Value=400  OutDataTypeStr=int32
  Constant2 : Constant  Value=440  OutDataTypeStr=int32
  Constant3 : Constant  OutDataTypeStr=int32
  Constant4 : Constant  OutDataTypeStr=int32
  Constant5 : Constant  OutDataTypeStr=int32
  Constant6 : Constant  Value=207  OutDataTypeStr=int32
  OutputScreenSwipe : Subsystem
  display_clear_screen : Raptor_display_lib/Drawing Functions/display_clear_screen  Priority=100  colorPort=off  l1Color=0000  l2Color=FFFF  pnPort=off
  display_draw_image : Raptor_display_lib/Drawing Functions/display_draw_image  imagePort=off  imageFile=top corner logo.png  opacityPort=off  opacity=100  drawMode=Draw Entire Image  alpha=Draw as Transparent  layer=Background  drawModeXY=Top Left  pnPort=off
  display_draw_image1 : Raptor_display_lib/Drawing Functions/display_draw_image  imagePort=off  imageFile=swipe_right_left.png  opacityPort=off  opacity=100  drawMode=Draw Entire Image  alpha=Draw as Transparent  layer=Foreground  drawModeXY=Top Left  pnPort=off
  display_draw_text : Raptor_display_lib/Drawing Functions/display_draw_text  textPort=off  textVal='Outputs'  colorPort=off  col=FFFF  opacity=100  font=Future  fontFile=''  heightPort=off  height=40  hAlign=Center  vAlign=Center  spacing=0  layer=Background  pnPort=off
  raptor_display_swipe_action2 : Raptor_display_lib/Touchscreen/raptor_display_swipe_action  gest_callback_sim_func_name='OutputScreenSwipe'
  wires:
  Constant6/1 -> display_draw_image1/1
  Constant5/1 -> display_draw_image1/2
  Constant3/1 -> display_draw_image/2
  Constant4/1 -> display_draw_image/1
  Constant16/1 -> display_draw_text/1
  Constant2/1 -> display_draw_text/2

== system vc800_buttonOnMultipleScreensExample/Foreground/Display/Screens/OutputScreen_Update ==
  function : TriggerPort  TriggerType=function-call  VariantControl=Variant
  OutputElement : Subsystem
  display_element1 : Raptor_display_lib/Drawing Functions/display_element  colorPort=off  col=0000  layer=Background  pnPort=off
  Actuators : Outport  VectorParamsAs1DForOutWhenUnconnected=off
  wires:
  display_element1/1 -> OutputElement/Trigger
  OutputElement/1(Out Bus Element1) -> Actuators/1
